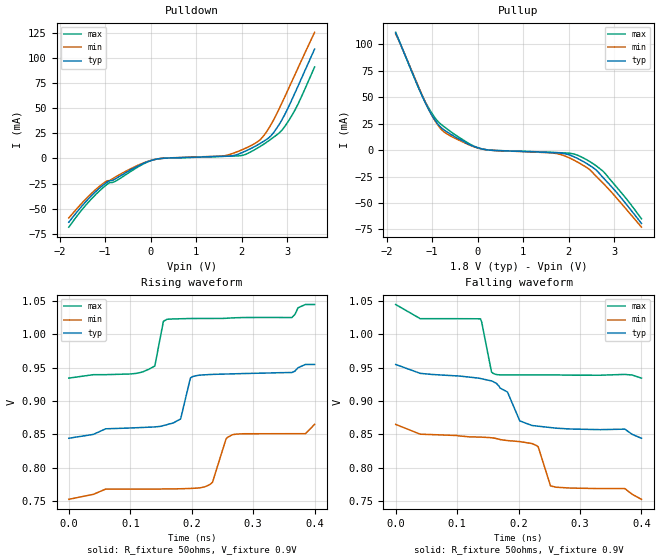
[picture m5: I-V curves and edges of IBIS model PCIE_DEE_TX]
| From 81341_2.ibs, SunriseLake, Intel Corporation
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[Model]   PCIE_DEE_TX
Model_type   Output
Polarity   Non-Inverting
|   typ   min   max
C_comp   0.14pF   0.126pF   0.154pF
[Voltage Range]   1.800V   1.620V   1.980V
[Temperature Range]   60.0   110.0   -5.0
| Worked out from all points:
|   slope of the pulldown table from 0 to 0.27 V, typ, clamps not added: 119 ohm
|   slope of the pullup table from 0 to 0.27 V, typ, clamps not added: 120 ohm
|   rising waveform, R_fixture 50ohms, V_fixture 0.9V: 20-80 % time 30.8ps typ, 25.8ps min, 20.4ps max; typ from 0.844 V to 0.955 V
|   falling waveform, R_fixture 50ohms, V_fixture 0.9V: 20-80 % time 70ps typ, 82.1ps min, 14.9ps max; typ from 0.955 V to 0.844 V
[Pulldown]
|   Voltage   I(typ)   I(min)   I(max)
-1.8V     -63.32mA   -59.07mA   -68.24mA
-1.44V    -43.57mA   -40.91mA   -47.09mA
-1.02V    -25.58mA   -23.94mA   -27.96mA
-60mV     -2.992mA   -2.787mA   -3.267mA
240mV     75.21uA    89.15uA    43.83uA
1.62V     2.24mA     2.69mA     2.13mA
2.04V     6.472mA    9.287mA    3.371mA
2.34V     13.24mA    16.36mA    10.18mA
2.64V     22.46mA    33.42mA    19.15mA
2.94V     43.2mA     60.75mA    31.48mA
3.24V     72.3mA     90.32mA    54.43mA
3.6V      108.7mA    125.3mA    90.91mA
[Pullup]
|   Voltage   I(typ)   I(min)   I(max)
-1.8V     110.5mA    109.7mA    111.3mA
-1.32V    61.33mA    62.07mA    61.04mA
-1.14V    43.81mA    44.44mA    44.62mA
-900mV    26.07mA    25.21mA    28.37mA
-720mV    18.5mA     16.59mA    21.54mA
-180mV    5.219mA    4.74mA     5.897mA
120mV     844.2uA    822.3uA    835uA
1.68V     -2.501mA   -2.942mA   -2.264mA
2.16V     -7.2mA     -10.54mA   -4.327mA
2.46V     -14.45mA   -18.48mA   -10.78mA
2.76V     -26.19mA   -31.48mA   -20.18mA
3.6V      -69.36mA   -72.88mA   -65.01mA
[Ramp]
| variable   typ   min   max
dV/dt_r   0.307/8.8859e-11 0.300/1.13715e-10 0.311/7.29426e-11
dV/dt_f   0.306/8.98485e-11 0.302/1.15352e-10 0.309/7.35806e-11
R_load = 50ohms
[Rising Waveform]
R_fixture = 50ohms
V_fixture = 0.9V
V_fixture_min = 0.81V
V_fixture_max = 0.99V
|   Time   V(typ)   V(min)   V(max)
0s        844.2mV    752.5mV    934.5mV
140ps     861.2mV    768mV      952.7mV
154ps     863.2mV    768mV      1.02V
160ps     864.7mV    768.1mV    1.023V
182ps     873.2mV    768.4mV    1.024V
202ps     936.9mV    769mV      1.024V
234ps     940.1mV    778.5mV    1.024V
256ps     940.6mV    843.4mV    1.024V
266ps     940.9mV    849.4mV    1.025V
400ps     955mV      865mV      1.045V
[Falling Waveform]
R_fixture = 50ohms
V_fixture = 0.9V
V_fixture_min = 0.81V
V_fixture_max = 0.99V
|   Time   V(typ)   V(min)   V(max)
0s        955mV      865mV      1.045V
40ps      941.6mV    850.3mV    1.024V
138ps     933.9mV    845.9mV    1.023V
156ps     930.3mV    844.9mV    943.5mV
162ps     927.6mV    844.1mV    940.3mV
182ps     913.6mV    840.7mV    939.3mV
202ps     870.3mV    839.2mV    939.3mV
232ps     862.3mV    831.2mV    939.3mV
252ps     860.3mV    772.6mV    939.3mV
400ps     844.2mV    752.5mV    934.5mV
